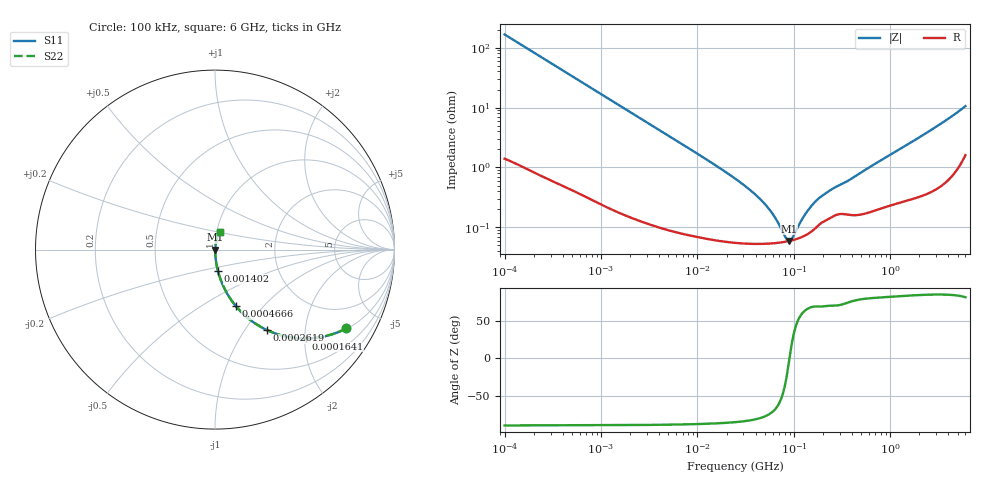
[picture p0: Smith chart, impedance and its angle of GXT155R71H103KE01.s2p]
!Murata Part Number: GXT155R71H103KE01
!These Parameters are Measured in Series Mode Connection
!Data Generated on Jan 08, 2026
!  o--ll--o
!Port1  Port2
!  o------o
!Operation Temp=25[degC], DC Bias Voltage=0[V]
!Freq. Start=100[kHz] Stop=6[GHz] 401[Steps]
# Hz S RI R 50
!Freq.(Hz) S11(Real) S11(Imag) S21(Real) S21(Imag) S12(Real) S12(Imag) S22(Real) S22(Imag)
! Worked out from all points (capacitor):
!   401 points, 100 kHz to 6 GHz, reference 50 ohm
!   read as one part in series: C = 9.59 nF near 105.7 kHz
!   lowest |Z| = 59.5 mohm at 89.23 MHz (marker M1)
!   series resonance near 89.98 MHz, so ESL is about 330 pH
!   S11 on the Smith chart (normalised r, x): 100 kHz: 1.03, -3.31; 164.1 kHz: 1.02, -2.03; 261.9 kHz: 1.01, -1.27; 466.6 kHz: 1.01, -0.72; 1.402 MHz: 1.00, -0.24; 6 GHz: 1.03, +0.21
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100000  0.7314 -0.439  0.2686 0.439  0.2686 0.439  0.7314 -0.439
164065  0.5066 -0.4952  0.4934 0.4952  0.4934 0.4952  0.5066 -0.4952
261871  0.2905 -0.4487  0.7095 0.4487  0.7095 0.4487  0.2905 -0.4487
466596  0.117 -0.3154  0.883 0.3154  0.883 0.3154  0.117 -0.3154
631452  0.0688 -0.2466  0.9312 0.2466  0.9312 0.2466  0.0688 -0.2466
1402027  0.0161 -0.1182  0.9839 0.1182  0.9839 0.1182  0.0161 -0.1182
3987316  0.0028 -0.0424  0.9972 0.0424  0.9972 0.0424  0.0028 -0.0424
2.517799e7  0.00059 -0.00632  0.9994 0.00632  0.9994 0.00632  0.00059 -0.00632
3.80366e7  0.000545 -0.00374  0.9995 0.00374  0.9995 0.00374  0.000545 -0.00374
5.147553e7  0.000539 -0.00226  0.9995 0.00226  0.9995 0.00226  0.000539 -0.00226
6.414516e7  0.000549 -0.00133  0.9995 0.00133  0.9995 0.00133  0.000549 -0.00133
8.216224e7  0.000578 -0.000351  0.9994 0.000351  0.9994 0.000351  0.000578 -0.000351
8.922949e7  0.000594 -3.21e-05  0.9994 3.21e-05  0.9994 3.21e-05  0.000594 -3.21e-05
9.690463e7  0.000613 0.000287  0.9994 -0.000287  0.9994 -0.000287  0.000613 0.000287
1.241232e8  0.000706 0.00126  0.9993 -0.00126  0.9993 -0.00126  0.000706 0.00126
1.546735e8  0.000876 0.00219  0.9991 -0.00219  0.9991 -0.00219  0.000876 0.00219
1.824266e8  0.00112 0.00288  0.9989 -0.00288  0.9989 -0.00288  0.00112 0.00288
2.401829e8  0.00146 0.00395  0.9985 -0.00395  0.9985 -0.00395  0.00146 0.00395
3.72965e8  0.00166 0.00591  0.9983 -0.00591  0.9983 -0.00591  0.00166 0.00591
9.76689e8  0.00253 0.0157  0.9975 -0.0157  0.9975 -0.0157  0.00253 0.0157
2.702311e9  0.00576 0.0426  0.9942 -0.0426  0.9942 -0.0426  0.00576 0.0426
6e9  0.0261 0.1  0.9739 -0.1  0.9739 -0.1  0.0261 0.1
